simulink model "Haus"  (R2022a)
settings: Solver=FixedStepAuto  StartTime=0.0  StopTime=T_Ende  FixedStep=T  MaxStep=T_max  RelTol=1e-3
libraries: EEZ_EnergieErzeugung x1, ESP_EnergieSpeicher x1, HZR_Heizungsregelung x1, HZT_Heizung_u_Klimatechnik x1, ISO_IsoliereigenschaftenHaus x1, LKT_Lastkollektive x1

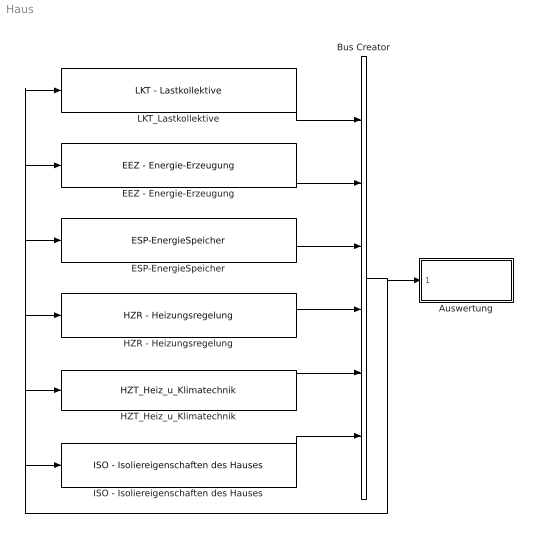
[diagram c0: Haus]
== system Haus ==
  Auswertung : Subsystem
  Bus Creator : BusCreator  Inputs=6
  EEZ - Energie-Erzeugung : EEZ_EnergieErzeugung/EEZ - Energie-Erzeugung  SystemSampleTime=-1  VariantActivationTime=update diagram  Latency=0  AutoFrameSizeCalculation=off
  ESP-EnergieSpeicher : ESP_EnergieSpeicher/ESP-EnergieSpeicher  SystemSampleTime=-1  VariantActivationTime=update diagram  Latency=0  AutoFrameSizeCalculation=off
  HZR - Heizungsregelung : HZR_Heizungsregelung/HZR - Heizungsregelung  SystemSampleTime=-1  VariantActivationTime=update diagram  Latency=0  AutoFrameSizeCalculation=off
  HZT_Heiz_u_Klimatechnik : HZT_Heizung_u_Klimatechnik/HZT_Heiz_u_Klimatechnik  SystemSampleTime=-1  VariantActivationTime=update diagram  Latency=0  AutoFrameSizeCalculation=off
  ISO - Isoliereigenschaften des Hauses : ISO_IsoliereigenschaftenHaus/ISO - Isoliereigenschaften des Hauses  SystemSampleTime=-1  VariantActivationTime=update diagram  Latency=0  AutoFrameSizeCalculation=off
  LKT_Lastkollektive : LKT_Lastkollektive/LKT - Lastkollektive  SystemSampleTime=-1  VariantActivationTime=update diagram  Latency=0  AutoFrameSizeCalculation=off
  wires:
  EEZ - Energie-Erzeugung/1 -> Bus Creator/2
  HZR - Heizungsregelung/1 -> Bus Creator/4
  LKT_Lastkollektive/1 -> Bus Creator/1
  Bus Creator/1 -> ISO - Isoliereigenschaften des Hauses/1, HZT_Heiz_u_Klimatechnik/1, LKT_Lastkollektive/1, EEZ - Energie-Erzeugung/1, ESP-EnergieSpeicher/1, HZR - Heizungsregelung/1, Auswertung/1(Eingang)
  ISO - Isoliereigenschaften des Hauses/1 -> Bus Creator/6
  HZT_Heiz_u_Klimatechnik/1 -> Bus Creator/5
  ESP-EnergieSpeicher/1 -> Bus Creator/3

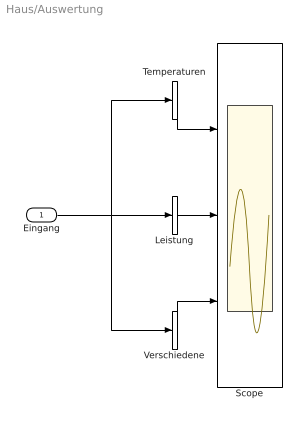
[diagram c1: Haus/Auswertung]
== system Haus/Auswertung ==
  Eingang : Inport
  Leistung : BusSelector  OutputSignals=HZT.HZT_Verbrauchteleistung,HZR.HZR_Warmwasserheizleistung_Waermepumpe,HZR.HZR_Warmwasserheizleistung,HZR.HZR_Heizleistung,HZT.HZT_Warmwasserspeicher_verbrauchte_Leistung,EEZ.EEZ_Warmwasserleistung,EEZ.EEZ_PVLeistungAC,ESP.ESP_Warmwassertemperatur  OutputAsBus=on
  Scope : Scope  NumInputPorts=3
  Temperaturen : BusSelector  OutputSignals=ISO.ISO_IstTemp,LKT.LKT_Temperatur,ESP.ESP_Warmwassertemperatur,HZR.HZR_Solltemperatur  OutputAsBus=on
  Verschiedene : BusSelector  OutputSignals=LKT.LKT_Stromverbrauch,LKT.LKT_Wasserverbrauch  OutputAsBus=on
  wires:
  Eingang/1 -> Verschiedene/1, Leistung/1, Temperaturen/1
  Temperaturen/1 -> Scope/1
  Leistung/1 -> Scope/2
  Verschiedene/1 -> Scope/3
